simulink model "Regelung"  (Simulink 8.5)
settings: Solver=ode45  StartTime=0.0  StopTime=25  MaxStep=0.5  MinStep=1e-2  RelTol=1e-3
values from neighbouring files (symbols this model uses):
  K = 'Error'    [berechneLQR.m]    (also in simGUI.m = str2num(get(h.reglerK, 'String')))
  stPendel = block.DialogPrm(1).Data    [systemPendel_V3.m]    (also in Versuch3.m = ladePendel(); simGUI.m = ladePendel(); Versuch4.m = ladePendel(); systemPendel_V5.m)
  x0 = block.DialogPrm(2).Data    [systemPendel_V3.m]    (also in Versuch3.m = [0.5 0 1*AP 0]; simGUI.m = [x1_0 x2_0 x3_0 x4_0]; Versuch4.m = [0.5 0 0 0]; systemPendel_V5.m)
  xArbeitspunkt = [0, 0, AP, 0]    [runPendel.m]

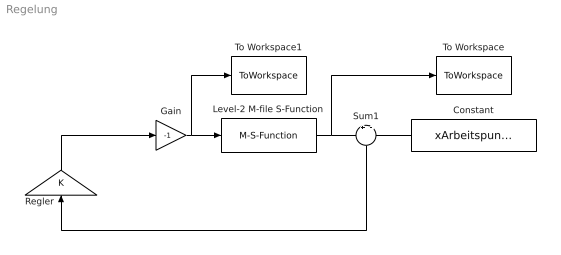
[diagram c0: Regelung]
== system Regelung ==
  Constant : Constant  Value=xArbeitspunkt
  Gain : Gain  Gain=-1
  Level-2 M-file S-Function : M-S-Function  FunctionName=systemPendel_V3  Parameters=stPendel,x0
  Regler : Gain  Gain=K  Multiplication=Matrix(K*u)
  Sum1 : Sum  Inputs=+|-
  To Workspace : ToWorkspace  VariableName=mZustand  SampleTime=-1
  To Workspace1 : ToWorkspace  VariableName=vInput  SampleTime=-1
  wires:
  Regler/1 -> Gain/1
  Level-2 M-file S-Function/1 -> Sum1/1, To Workspace/1
  Constant/1 -> Sum1/2
  Sum1/1 -> Regler/1
  Gain/1 -> To Workspace1/1, Level-2 M-file S-Function/1
